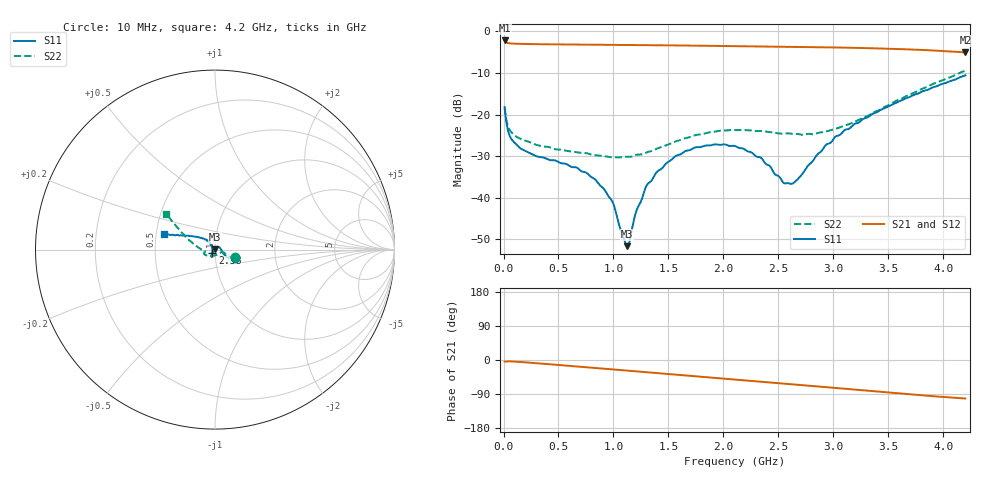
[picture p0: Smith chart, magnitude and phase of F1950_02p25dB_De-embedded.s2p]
! Integrated Device Technology
! Corporate Headquarters
! 6024 Silver Creek Valley Road
! San Jose, CA 95138  USA
! Phone:  1-408-284-8200
! Toll Free:  1-800-223-1366
! Webpage:  http://www.idt.com/
! Timing and RF Division
! 515 Groton Road, Suite 102
! Westford, MA 01886-6024
! Device:  F1950
! Description: 7-bit 0.25 dB Digital Step Attenuator
! Frequency:  150.0 -  4000.00 MHz
! Package:  4x4 mm Thin QFN Plastic Package: 24 pin
! Ports:  2 RF, 12 DC
!  Pin  1  = D0
!  Pin  2  = VDD
!  Pin  3  = Vmode
!  Pin  4  = GND
!  Pin  5  = RF1  =  Port 1
!  Pin  6  = GND
!  Pin  7  = GND
!  Pin  8  = GND
!  Pin  9  = GND
!  Pin 10  = GND
!  Pin 11  = GND
!  Pin 12  = GND
!  Pin 13  = GND
!  Pin 14  = RF2  =  Port 2
!  Pin 15  = GND
!  Pin 16  = LE
!  Pin 17  = CLK
!  Pin 18  = DATE
!  Pin 19  = D6
!  Pin 20  = D5
!  Pin 21  = D4
!  Pin 22  = D3
!  Pin 23  = D2
!  Pin 24  = D1
! State:  9
! Atten State:  2.25 dB
! Voltage:  +5.00 Volts
! Current:  Not Measured mA
! Data:  The device was measured on a the F195X evaluation board which has
!  individual transmission lines to the RF pins.  Data was collected
!  using a calibrated network analyzer.  The evaluation board was
!  de-embedded using a TRL calibration technique.
!  The reference plane is the edge of the package pin.
! Misc:  Board 2019
!  Action Tracker AT0250
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# GHz S dB R 50
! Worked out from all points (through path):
!   420 points, 10 MHz to 4.2 GHz, reference 50 ohm
!   highest |S21| = -2.17 dB at 10 MHz (marker M1); lowest = -5.1 dB at 4.2 GHz (marker M2)
!   group delay of S21, straight-line fit = 67 ps
!   lowest |S11| = -51.6 dB at 1.12 GHz (marker M3), VSWR 1.01, Z = 49.8 + j0.101 ohm
!   |S11| at or under -10 dB: start of sweep to end of sweep
!   |S22| runs from -30.3 to -9.4 dB; largest |S21 - S12| = 0.00088
!   S11 on the Smith chart (normalised r, x): 10 MHz: 1.25, -0.12; 2.38 GHz: 0.97, -0.04; 4.2 GHz: 0.55, +0.11
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0.01  -18.16 -22.5  -2.17 -3.9  -2.17 -3.9  -18.38 -20.3
0.06  -25.32 -26.4  -2.87 -3.6  -2.87 -3.6  -23.84 -23.7
0.15  -28.06 -12.9  -2.99 -5.1  -2.99 -5.1  -25.77 -18.8
0.71  -33.65 45.9  -3.17 -18.1  -3.17 -18.1  -29.20 -31.2
0.84  -35.79 55.0  -3.19 -21.2  -3.19 -21.2  -29.77 -41.4
0.98  -40.45 66.0  -3.23 -24.5  -3.22 -24.5  -30.27 -57.4
1.12  -51.63 157.1  -3.26 -27.9  -3.26 -27.9  -30.14 -77.4
1.14  -51.11 -178.5  -3.26 -28.3  -3.26 -28.3  -30.15 -80.8
1.2  -43.86 -150.1  -3.27 -29.8  -3.27 -29.8  -29.70 -89.6
1.29  -37.69 -133.8  -3.29 -31.9  -3.29 -31.9  -29.23 -102.8
1.41  -33.45 -126.4  -3.32 -34.8  -3.32 -34.8  -28.04 -117.7
1.57  -29.90 -122.6  -3.37 -38.6  -3.36 -38.7  -26.39 -132.8
1.74  -27.91 -120.1  -3.41 -42.7  -3.41 -42.8  -24.97 -144.0
2.11  -27.60 -117.8  -3.53 -51.7  -3.52 -51.7  -23.73 -158.6
2.38  -31.72 -126.0  -3.62 -58.1  -3.61 -58.1  -24.06 -163.3
2.55  -36.49 -155.1  -3.66 -62.2  -3.66 -62.2  -24.56 -166.6
2.61  -36.62 -177.7  -3.68 -63.7  -3.68 -63.7  -24.57 -166.5
2.67  -35.68 157.7  -3.70 -65.1  -3.70 -65.2  -24.65 -167.2
2.81  -31.23 132.0  -3.76 -68.6  -3.76 -68.6  -24.73 -170.5
3.1  -23.75 130.2  -3.90 -75.8  -3.89 -75.9  -22.69 -178.8
3.51  -17.89 145.8  -4.16 -86.0  -4.16 -86.1  -17.66 163.5
4.2  -10.57 162.9  -5.06 -101.5  -5.05 -101.6  -9.45 143.6
